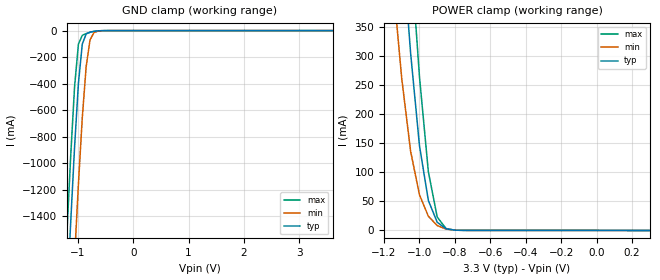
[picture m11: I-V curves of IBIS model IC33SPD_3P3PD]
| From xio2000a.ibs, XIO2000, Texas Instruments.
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|   Model IC33SPD_3P3PD
[Model]   IC33SPD_3P3PD
Model_type   Input
Polarity   Non-Inverting
Vinl =   0.9900V
Vinh =   2.3100V
C_comp   2.1080pF   2.1980pF   2.1240pF
[Model Spec]
|   typ   min   max
Vinh   2.31V   2.10V   2.52V
Vinl   0.99V   0.90V   1.08V
[Temperature Range]   25.0000   0.1250k   -40.0000
[Voltage Range]   3.3000V   3.0000V   3.6000V
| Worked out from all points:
|   GND clamp passes 1 mA (typ) near -0.59 V on its own axis
|   POWER clamp passes 1 mA (typ) near -0.81 V on its own axis
| (Vdd votage range)   1.50V   1.35V   1.65V
| (Process strength)   nominal   weak   strong
[GND_clamp]
| voltage   I(typ)   I(min)   I(max)
-3.3V     -22.44A    -23.23A    -22.01A
-1.2V     -2.062A    -2.938A    -1.55A
-1.13V    -1.453A    -2.319A    -952.1mA
-1.06V    -884.3mA   -1.722A    -427mA
-990mV    -399.1mA   -1.159A    -102.3mA
-920mV    -102mA     -657.3mA   -35.77mA
-850mV    -24.71mA   -270.7mA   -22.5mA
-780mV    -11.53mA   -70.04mA   -13.06mA
-710mV    -5.708mA   -15.33mA   -5.945mA
-640mV    -2.201mA   -4.331mA   -1.849mA
3.6V      0A         0A         0A
[POWER_clamp]
| voltage   I(typ)   I(min)   I(max)
-3.3V     12.64A     11.74A     13.39A
-1.15V    732.8mA    427.9mA    979.8mA
-1.1V     506.3mA    260.6mA    722.9mA
-1.05V    304.3mA    136mA      480.2mA
-1V       145.6mA    61.08mA    263.9mA
-950mV    51.64mA    24.48mA    101.1mA
-900mV    14.1mA     8.434mA    23.11mA
-850mV    2.893mA    2.41mA     3.321mA
-800mV    542.9uA    638.7uA    481.2uA
-750mV    166.7uA    192uA      208uA
300mV     0A         0A         0A
